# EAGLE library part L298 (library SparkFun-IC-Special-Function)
L298 Dual Full Bridge Driver
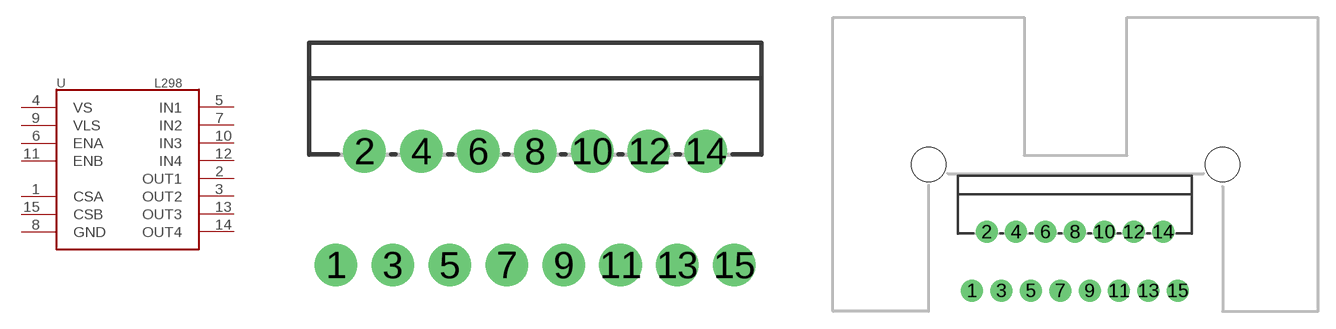
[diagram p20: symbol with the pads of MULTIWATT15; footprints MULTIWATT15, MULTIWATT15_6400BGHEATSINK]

Designator prefix U

## L298  [MULTIWATT15]
1  CSA
2  OUT1
3  OUT2
4  VS
5  IN1
6  ENA
7  IN2
8  GND
9  VLS
10  IN3
11  ENB
12  IN4
13  OUT3
14  OUT4
15  CSB

## L298HEATSINK  [MULTIWATT15_6400BGHEATSINK]
Pads as for MULTIWATT15

## Footprint MULTIWATT15 (pad centres in mm)
Multiwatt15V package for the L298 dual full bridge driver
drill 1.1 pad 1.9: 1 -8.95,-2.39; 2 -7.68,2.69; 3 -6.41,-2.39; 4 -5.14,2.69; 5 -3.87,-2.39; 6 -2.6,2.69; 7 -1.33,-2.39; 8 -0.06,2.69; 9 1.21,-2.39; 10 2.48,2.69; 11 3.75,-2.39; 12 5.02,2.69; 13 6.29,-2.39; 14 7.56,2.69; 15 8.83,-2.39

## Footprint MULTIWATT15_6400BGHEATSINK (pad centres in mm)
drill 1.1 pad 1.9: 1 -8.95,-2.39; 2 -7.68,2.69; 3 -6.41,-2.39; 4 -5.14,2.69; 5 -3.87,-2.39; 6 -2.6,2.69; 7 -1.33,-2.39; 8 -0.06,2.69; 9 1.21,-2.39; 10 2.48,2.69; 11 3.75,-2.39; 12 5.02,2.69; 13 6.29,-2.39; 14 7.56,2.69; 15 8.83,-2.39
hole 2.997 at -12.7,8.509
hole 2.997 at 12.7,8.509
